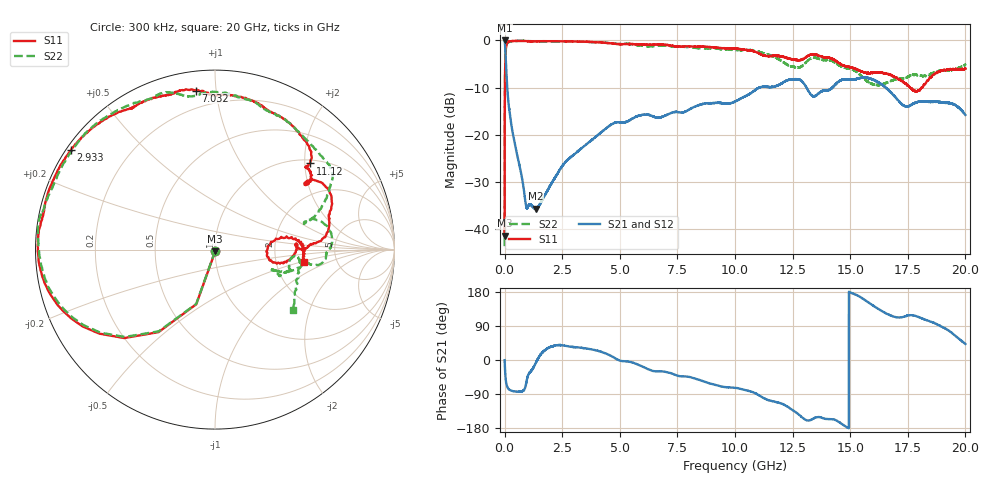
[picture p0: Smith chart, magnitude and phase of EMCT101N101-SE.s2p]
!EMCT101N101
!Johanson Technology Inc.
!www.johansontechnology.com
!Test Board Conditions:
!Substrate Type  RO4350B
!Substrate Thickness  10 mil
!Substrate Dk  3.66
!TL Type: GCPW
!TL Trace Width  22 mil
!TL Gap  14 mil
!PART MODE SINGLE ENDED (AKA BYPASS)
!DUT TOPOLOGY	SERIES-SHUNT
# MHz S  dB  R 50
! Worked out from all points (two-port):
!   20001 points, 300 kHz to 20 GHz, reference 50 ohm
!   highest |S21| = -0.01 dB at 1.3 MHz (marker M1); lowest = -35.6 dB at 1.356 GHz (marker M2)
!   |S21| within 3 dB of the highest: start of sweep to 38.44 MHz
!   lowest |S11| = -41.4 dB at 300 kHz (marker M3), VSWR 1.02, Z = 50.2 - j0.841 ohm
!   |S11| at or under -10 dB: start of sweep to 13.06 MHz; 17.6 GHz to 18.12 GHz (523.2 MHz wide, 2.93 % of centre)
!   |S22| runs from -43.6 to 0.0 dB; largest |S21 - S12| = 0.0099
!   S11 on the Smith chart (normalised r, x): 300 kHz: 1.00, -0.02; 2.933 GHz: 0.01, +0.31; 7.032 GHz: 0.10, +0.88; 11.12 GHz: 1.08, +2.12; 20 GHz: 2.89, -0.55
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0.3  -41.38 -79.4  -0.02 -0.4  0.01 -0.6  -43.57 -80.8
1.3  -29.55 -90.5  -0.01 -1.9  -0.01 -2.0  -29.69 -90.5
101.298  -0.67 -160.1  -9.04 -68.6  -9.00 -68.6  -0.76 -160.4
134.298  -0.42 -165.3  -11.29 -73.2  -11.23 -73.3  -0.51 -165.5
326.295  -0.14 -176.1  -18.86 -81.6  -18.83 -81.8  -0.21 -177.4
920.286  -0.14 172.9  -34.74 -66.4  -34.85 -66.5  -0.05 169.7
1356.28  -0.20 167.3  -35.64 -7.5  -35.58 -7.1  -0.18 164.4
2933.256  -0.20 145.2  -24.50 34.6  -24.50 34.3  -0.28 141.9
3334.25  -0.26 140.2  -22.85 32.1  -22.86 32.2  -0.27 136.0
4752.229  -0.70 122.4  -17.48 6.3  -17.51 6.3  -0.67 117.0
6667.2  -0.85 102.5  -16.39 -29.8  -16.36 -30.0  -1.15 93.5
7032.195  -0.99 96.8  -15.80 -31.9  -15.81 -32.1  -1.16 86.8
10000.15  -1.73 60.6  -12.94 -73.3  -12.78 -73.7  -2.01 45.9
11120.13  -2.92 42.2  -9.88 -96.0  -10.01 -95.8  -2.54 29.7
12703.11  -4.17 35.7  -8.23 -140.6  -8.19 -140.6  -5.76 16.4
13334.1  -2.96 29.0  -11.67 -157.0  -11.64 -157.3  -3.75 9.0
14397.08  -4.42 5.6  -9.14 -159.4  -9.20 -159.0  -4.89 -8.6
15456.07  -6.52 0.4  -7.96 165.6  -7.85 165.2  -7.45 -16.5
16667.05  -7.17 -4.4  -10.55 119.7  -10.65 120.2  -8.75 -20.1
17851.03  -10.78 -2.9  -13.14 115.9  -12.96 116.8  -7.20 -15.6
18685.02  -7.00 7.6  -12.99 96.6  -12.88 96.3  -6.76 -4.9
20000  -5.99 -8.2  -15.79 42.3  -15.97 43.7  -5.17 -37.6
